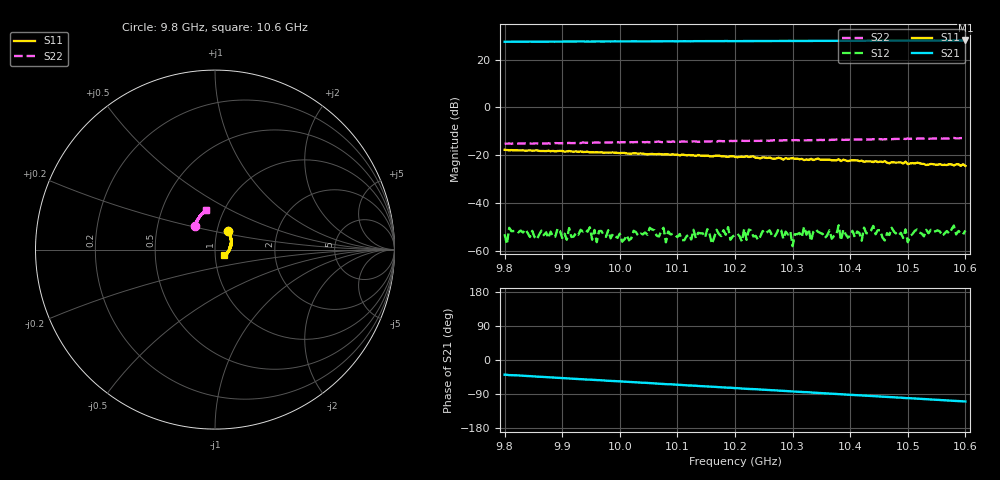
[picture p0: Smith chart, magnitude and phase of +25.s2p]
!Agilent Technologies,E8361C,US49010292,A.09.42.06
!Agilent E8361C: A.09.42.06
!Date: Tuesday, October 15, 2024 21:36:08
!Correction: S11(Full 2 Port(1,2))
!S21(Full 2 Port(1,2))
!S12(Full 2 Port(1,2))
!S22(Full 2 Port(1,2))
!S2P File: Measurements: S11, S21, S12, S22:
# Hz S  dB  R 50
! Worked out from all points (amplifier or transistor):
!   201 points, 9.8 GHz to 10.6 GHz, reference 50 ohm
!   highest |S21| = 28.0 dB at 10.6 GHz (marker M1)
!   |S21| within 3 dB of that: start of sweep to end of sweep
!   unconditionally stable (mu >= 1): start of sweep to end of sweep
!   at 9.932 GHz: K = 7.48, MAG = 27.7 dB, |S12| = -51.3 dB
!   at 10.2 GHz: K = 9.31, MAG = 27.9 dB, |S12| = -53.5 dB
!   at 10.6 GHz: K = 7.22, MAG = 28.2 dB, |S12| = -51.6 dB
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9.8e9  -17.83 55.3  27.43 -38.8  -53.19 49.6  -15.27 131.1
9.804e9  -17.89 55.0  27.43 -39.1  -57.39 49.5  -15.25 131.1
9.808e9  -17.99 53.5  27.45 -39.9  -50.50 67.9  -15.23 131.7
9.824e9  -18.07 52.5  27.49 -40.7  -52.39 40.5  -15.23 130.2
9.932e9  -18.48 42.9  27.51 -50.4  -51.35 46.6  -15.02 125.8
9.936e9  -18.74 43.0  27.60 -51.0  -52.08 50.7  -14.77 125.4
9.948e9  -18.91 42.3  27.51 -51.7  -50.24 27.1  -14.92 126.3
9.96e9  -18.80 41.7  27.57 -53.0  -56.49 45.4  -14.73 125.4
9.98e9  -19.00 39.4  27.59 -54.9  -51.47 45.0  -14.74 124.5
1.0004e10  -19.11 35.2  27.60 -56.8  -56.29 25.0  -14.66 124.1
1.0068e10  -19.55 30.6  27.64 -62.3  -54.16 57.9  -14.36 122.0
1.02e10  -20.74 16.8  27.70 -74.2  -53.48 43.8  -14.11 117.9
1.0276e10  -21.15 8.7  27.75 -80.8  -50.74 42.3  -13.94 114.9
1.0296e10  -21.47 5.7  27.79 -82.8  -52.00 42.5  -13.88 114.3
1.03e10  -21.27 6.8  27.74 -82.9  -58.18 45.7  -13.81 114.1
1.032e10  -22.14 2.4  27.77 -84.8  -50.07 45.2  -13.85 114.5
1.0332e10  -21.60 -0.5  27.82 -85.8  -56.11 35.4  -13.82 113.3
1.0336e10  -22.09 -0.5  27.78 -86.1  -52.18 43.3  -13.76 113.9
1.0432e10  -22.70 -8.9  27.90 -94.8  -52.59 21.3  -13.45 109.3
1.0468e10  -23.44 -17.6  27.88 -97.8  -53.48 45.5  -13.30 108.4
1.0524e10  -23.70 -21.3  27.95 -102.7  -52.84 15.3  -13.08 105.9
1.06e10  -24.57 -30.7  27.98 -109.5  -51.61 31.0  -12.88 102.8
